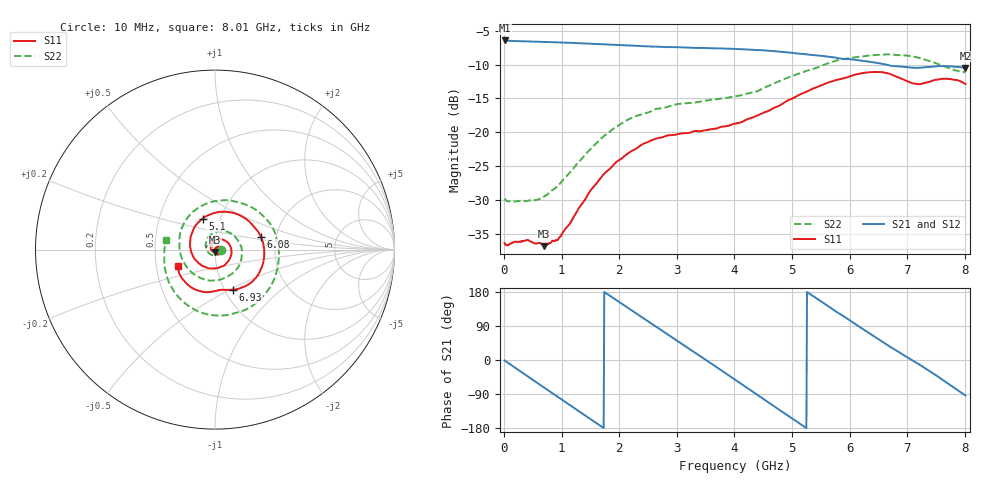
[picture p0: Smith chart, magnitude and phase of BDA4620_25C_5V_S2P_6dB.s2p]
!Agilent Technologies,E5071B,MY42404982,A.09.10
!Date: Wed May 06 08:59:22 2026
!Data & Calibration Information:
!Freq	S11:SOLT2(ON)	S21:SOLT2(ON)	S12:SOLT2(ON)	S22:SOLT2(ON)
# Hz S RI R 50
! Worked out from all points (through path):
!   801 points, 10 MHz to 8.01 GHz, reference 50 ohm
!   highest |S21| = -6.44 dB at 10 MHz (marker M1); lowest = -10.5 dB at 8.01 GHz (marker M2)
!   group delay of S21, straight-line fit = 282 ps
!   lowest |S11| = -36.9 dB at 700 MHz (marker M3), VSWR 1.03, Z = 50.1 - j1.43 ohm
!   |S11| at or under -10 dB: start of sweep to end of sweep
!   |S22| runs from -30.3 to -8.5 dB; largest |S21 - S12| = 0.0019
!   S11 on the Smith chart (normalised r, x): 10 MHz: 1.03, -0.00; 5.1 GHz: 0.82, +0.30; 6.08 GHz: 1.66, +0.26; 6.93 GHz: 1.09, -0.52; 8.01 GHz: 0.65, -0.12
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1e7  0.0151 -0.000913  0.4763 -0.0102  0.4769 -0.0101  0.0323 -0.00245
3.3e8  0.0134 -0.00813  0.386 -0.2679  0.3866 -0.2686  0.0205 -0.0231
7e8  0.00134 -0.0143  0.1338 -0.4451  0.134 -0.4457  -0.0121 -0.0312
1.01e9  -0.016 -0.00782  -0.1218 -0.4433  -0.1221 -0.4438  -0.0426 -0.00995
1.35e9  -0.0246 0.0162  -0.3501 -0.2889  -0.3501 -0.2891  -0.0507 0.0386
1.65e9  -0.0128 0.0423  -0.4423 -0.0679  -0.4428 -0.0681  -0.0235 0.0833
1.94e9  0.0155 0.0574  -0.4127 0.1575  -0.4137 0.1582  0.0311 0.1045
2.32e9  0.0611 0.0466  -0.2184 0.3755  -0.2192 0.3758  0.1101 0.0741
2.68e9  0.0907 0.00384  0.0451 0.4255  0.0456 0.4258  0.1491 -0.00276
3e9  0.0841 -0.047  0.2644 0.3327  0.2646 0.3326  0.1358 -0.0866
3.39e9  0.0392 -0.0938  0.411 0.0869  0.4115 0.0861  0.0484 -0.1604
3.69e9  -0.0143 -0.1056  0.3943 -0.1341  0.3941 -0.1351  -0.051 -0.1679
4.01e9  -0.0765 -0.0864  0.2551 -0.324  0.2548 -0.3246  -0.1498 -0.107
4.52e9  -0.1388 0.0173  -0.1008 -0.3893  -0.1013 -0.3898  -0.1951 0.0864
5.1e9  -0.0691 0.1732  -0.3674 -0.1035  -0.3681 -0.1026  -0.00468 0.2695
5.35e9  0.0134 0.2085  -0.3667 0.0625  -0.367 0.0632  0.1204 0.2658
5.73e9  0.1583 0.1803  -0.237 0.2674  -0.2369 0.2681  0.2901 0.1651
6.08e9  0.2551 0.0725  -0.04 0.3411  -0.0392 0.3417  0.3564 -0.0224
6.68e9  0.1938 -0.1897  0.2496 0.1874  0.2507 0.1875  0.1985 -0.3193
6.93e9  0.1 -0.224  0.2955 0.0723  0.2966 0.0712  0.057 -0.3657
7.48e9  -0.0536 -0.2369  0.2402 -0.1888  0.2404 -0.1899  -0.2299 -0.2304
8.01e9  -0.2088 -0.0904  -0.0187 -0.298  -0.0192 -0.2991  -0.2713 0.0536
